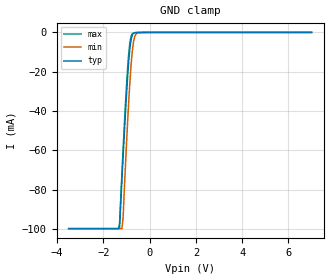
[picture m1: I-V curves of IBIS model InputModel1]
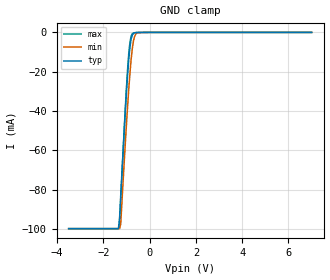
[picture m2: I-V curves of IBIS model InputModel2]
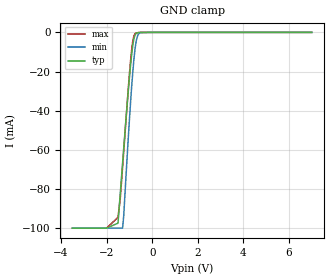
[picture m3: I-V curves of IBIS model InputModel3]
[IBIS Ver]   2.1
[File name]   e_200bv3.ibs   | e_= TSOP, f200bv= abbr chip name, 3= 3.3V Vcc
[File Rev]   2.00
[Date]   13-March-1996
[Source]   File generated from lab measurements at Intel Corporation
[Notes]   Rev 2.00 All data was replaced by actual measurements
   performed in a lab.
[Disclaimer] INTEL DEVELOPER'S SOFTWARE LICENSE AGREEMENT
| BY USING THIS SOFTWARE, YOU ARE AGREEING TO BE BOUND
| BY THE TERMS OF THIS AGREEMENT.  DO NOT USE THE SOFTWARE
| UNTIL YOU HAVE CAREFULLY READ AND AGREED TO THE FOLLOWING
| TERMS AND CONDITIONS.  IF YOU DO NOT AGREE TO THE TERMS
| OF THIS AGREEMENT, PROMPTLY RETURN THE SOFTWARE PACKAGE
| AND ANY ACCOMPANYING ITEMS.
| IF YOU USE THIS SOFTWARE, YOU WILL BE BOUND BY THE TERMS
| OF THIS AGREEMENT
| LICENSE: Intel Corporation ("Intel") grants you the non-exclusive right
| to use the enclosed software program ("Software").  You will not use,
| copy, modify, rent, sell or transfer the Software or any portion
| thereof, except as provided in this Agreement.
| System OEM Developers may:
| 1.   Copy the Software for support, backup or archival purposes;
| 2.   Install, use, or distribute Intel owned Software in object code
|   only;
| 3.   Modify and/or use Software source code that Intel directly makes
|   available to you as an OEM Developer;
| 4.   Install, use, modify, distribute, and/or make or have made
|   derivatives ("Derivatives") of Intel owned Software under the
|   terms and conditions in this Agreement, ONLY if you are a System
|   OEM Developer and NOT an end-user.
| RESTRICTIONS:
| YOU WILL NOT:
| 1.   Copy the Software, in whole or in part, except as provided for
|   in this Agreement;
| 2.   Decompile or reverse engineer any Software provided in object
|   code format;
| 3.   Distribute any Software or Derivative code to any end-users,
|   unless approved by Intel in a prior writing.
| TRANSFER: You may transfer the Software to another OEM
| Developer if the receiving party agrees to the terms of this
| Agreement at the sole risk of any receiving party.
| OWNERSHIP AND COPYRIGHT OF SOFTWARE:
| Title to the Software and all copies thereof remain with Intel
| or its vendors.  The Software is copyrighted and is protected by
| United States and international copyright laws.  You will not
| remove the copyright notice from the Software.  You agree to
| prevent any unauthorized copying of the Software.
| DERIVATIVE WORK: OEM Developers that make or have made
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[Copyright]   Copyright 1996, Intel Corporation, All Rights Reserved
[Component]   E28F200BV   | 56-lead TSOP package, 28F200BV
[Manufacturer]  Intel   | Boot Block (tm)
|   | operating in 3.3V Vcc range
[Package]
|Variable   typ   min   max
|The following values apply for the Copper leadframe.
R_pkg   48m   41m   54m
L_pkg   4.92nH   4.44nH   5.39nH
C_pkg   0.48pF   0.45pF   0.50pF
|The following values apply for the Alloy-42 leadframe.
|R_pkg   195m   180m   210m
|L_pkg   4.92nH   4.44nH   5.39nH
|C_pkg   0.48pF   0.45pF   0.50pF
|*****************************Pin Definitions*****************************
[Pin]   signal_name   model_name   R_pin   L_pin   C_pin
 1   NC   InputModel4
 2   NC   InputModel4
 3   A15   InputModel3
 4   A14   InputModel3
 5   A13   InputModel3
 6   A12   InputModel3
 7   A11   InputModel3
 8   A10   InputModel3
 9   A09   InputModel1
10   A08   InputModel1
11   NC   InputModel4
12   NC   InputModel4
13   WE#   InputModel1
14   RP#   InputModel1
15   NC   InputModel4
16   NC   InputModel4
17   VPP   POWER
18   WP#   InputModel1
19   NC   InputModel4
20   NC   InputModel3
21   A07   InputModel3
22   A06   InputModel3
23   A05   InputModel3
24   A04   InputModel3
25   A03   InputModel3
26   A02   InputModel3
27   A01   InputModel3
28   NC   InputModel3
29   NC   InputModel4
30   NC   InputModel4
31   A00   InputModel2
32   CE#   InputModel1
33   GND   GND
34   OE#   InputModel1
35   DQ0   InputOutput
36   DQ8   InputOutput
37   DQ1   InputOutput
38   DQ9   InputOutput
39   DQ2   InputOutput
40   DQ10   InputOutput
41   DQ3   InputOutput
42   DQ11   InputOutput
43   VCC   POWER
44   VCC   POWER
45   DQ4   InputOutput
46   DQ12   InputOutput
47   DQ5   InputOutput
48   DQ13   InputOutput
49   DQ6   InputOutput
50   DQ14   InputOutput
51   DQ7   InputOutput
52   DQ15   InputOutput
53   GND   GND
54   BYTE#   InputModel2
55   A16   InputModel2
56   NC   InputModel4
|***********************Input Model 4******************************
[Model]   InputModel4
Model_type   Input
|   Model for all NC pins, excluding NC pin #20.
Vinl = 0.8V
Vinh = 2.0V
|Variable   Typ   Min   Max
C_comp   5.61p   NA   7.6p
[Voltage Range]   3.3V   3.0V   3.6V
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| Models and submodels in the file (5): InputModel1 (Input), InputModel2 (Input), InputModel3 (Input), InputModel4 (Input), InputOutput (I/O)
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|*********************Input Model 1************************************
[Model]   InputModel1
Model_type   Input
|   Model for WE#, WP#, RP#, OE# & CE#.
Vinl = 0.8V
Vinh = 2.0V
|Variable   Typ   Min   Max
C_comp   5.61p   NA   7.6p
[Voltage Range]   3.3V   3.0V   3.6V
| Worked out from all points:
|   GND clamp passes 1 mA (typ) near -0.73 V on its own axis
[GND_clamp]
|Voltage  I(typ)   I(min)   I(max)
-3.5V     -99.85mA   -99.85mA   -99.85mA
-1.35V    -99.85mA   -99.85mA   -99.85mA
-1.3V     -99.26mA   -99.85mA   -97.14mA
-1.2V     -75.18mA   -99.85mA   -72.14mA
-1.15V    -63.89mA   -94.76mA   -60.07mA
-1V       -31.6mA    -56.54mA   -27.07mA
-900mV    -14.05mA   -34.26mA   -10.17mA
-850mV    -7.687mA   -24.68mA   -4.745mA
-750mV    -1.284mA   -9.549mA   -630.3uA
-650mV    -225.8uA   -2.279mA   -169.1uA
-500mV    -29.1uA    -152uA     -20.31uA
7V        0A         0A         0A
[Power_clamp]
| Input buffer circuits of this product do not intrinsically
| require a [Power_clamp] definition.  This zero current
| [Power_clamp] table is provided for the compatibility with
| some IBIS parsers.
|Voltage  I(typ)   I(min)   I(max)
-3.3V     0A         0A         0A
0V        0A         0A         0A
3.3V      0A         0A         0A
7V        0A         0A         0A
|*********************Input Model 2******************************
[Model]   InputModel2
Model_type   Input
|   Model for A[0], A[16] & BYTE# pins.
Vinl = 0.8V
Vinh = 2.0V
|Variable   Typ   Min   Max
C_comp   5.61p   NA   7.6p
[Voltage Range]   3.3V   3.0V   3.6V
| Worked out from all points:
|   GND clamp passes 1 mA (typ) near -0.73 V on its own axis
[GND_clamp]
|Voltage  I(typ)   I(min)   I(max)
-3.5V     -99.85mA   -99.83mA   -99.85mA
-1.35V    -99.85mA   -99.83mA   -99.85mA
-1.3V     -94.37mA   -99.83mA   -98.64mA
-1.25V    -82.89mA   -97.51mA   -85.83mA
-1.1V     -50.15mA   -66.04mA   -49.42mA
-950mV    -21.04mA   -36.93mA   -18.24mA
-900mV    -13.36mA   -28.31mA   -10.32mA
-850mV    -7.565mA   -20.57mA   -4.846mA
-750mV    -1.296mA   -8.199mA   -639.8uA
-650mV    -228.2uA   -2.043mA   -174.9uA
-500mV    -30.35uA   -138.9uA   -20.97uA
7V        0A         0A         0A
[Power_clamp]
| Input buffer circuits of this product do not intrinsically
| require a [Power_clamp] definition.  This zero current
| [Power_clamp] table is provided for the compatibility with
| some IBIS parsers.
|Voltage  I(typ)   I(min)   I(max)
-3.3V     0A         0A         0A
0V        0A         0A         0A
3.3V      0A         0A         0A
7V        0A         0A         0A
|***********************Input Model 3******************************
[Model]   InputModel3
Model_type   Input
|   Model for A[15:1] & NC pin #20.
Vinl = 0.8V
Vinh = 2.0V
|Variable   Typ   Min   Max
C_comp   5.61p   NA   7.6p
[Voltage Range]   3.3V   3.0V   3.6V
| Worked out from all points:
|   GND clamp passes 1 mA (typ) near -0.73 V on its own axis
[GND_clamp]
|Voltage  I(typ)   I(min)   I(max)
-3.5V     -99.85mA   -99.85mA   -99.84mA
-2V       -99.85mA   -99.85mA   -99.84mA
-1.5V     -97.31mA   -99.85mA   -94.31mA
-1.4V     -82.07mA   -99.85mA   -84.51mA
-1.3V     -66.84mA   -99.85mA   -68.9mA
-1.25V    -59.17mA   -93.69mA   -60.87mA
-950mV    -16.82mA   -35.79mA   -14.52mA
-850mV    -6.51mA    -20.05mA   -4.331mA
-750mV    -1.251mA   -8.08mA    -628.9uA
-650mV    -222.2uA   -2.03mA    -171.1uA
-500mV    -30.37uA   -137.4uA   -20.58uA
7V        0A         0A         0A
[Power_clamp]
| Input buffer circuits of this product do not intrinsically
| require a [Power_clamp] definition.  This zero current
| [Power_clamp] table is provided for the compatibility with
| some IBIS parsers.
|Voltage  I(typ)   I(min)   I(max)
-3.3V     0A         0A         0A
0V        0A         0A         0A
3.3V      0A         0A         0A
7V        0A         0A         0A
